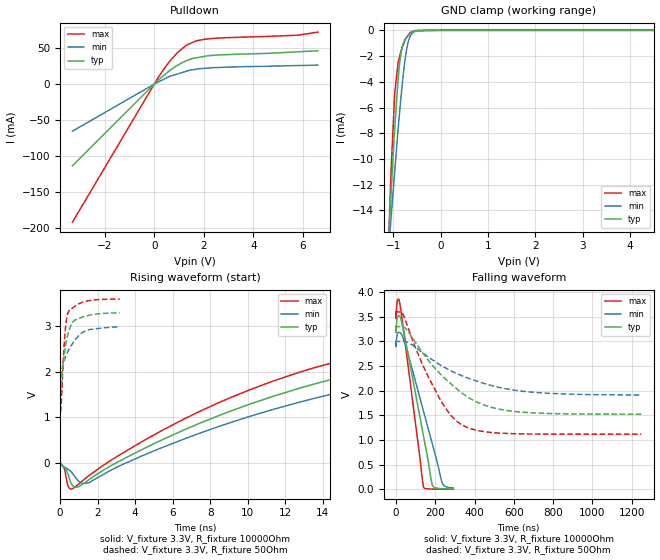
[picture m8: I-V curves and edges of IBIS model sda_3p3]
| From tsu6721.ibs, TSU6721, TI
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|   sda_3p3 Model
[Model]   sda_3p3
Model_type   I/O_open_drain
Polarity   Non-Inverting
Enable   Active-High
Vinl = 0.99
Vinh = 2.31
Vmeas = 1.65
Vref = 3.3
Cref = 35pF
Rref = 10000
|   typ   min   max
C_comp   1.333e-12   1.174e-12   1.472e-12
[Model spec]
Vinl   0.99   0.9   1.08
Vinh   2.31   2.1   2.52
[Voltage Range]   3.3   3   3.6
|Ambient Temperature   25   85   -40
|Junction Temperature
[Temperature Range]   27   125   -40
[Pullup Reference]   3.3   3   3.6
[Pulldown Reference]   0   0   0
[Power Clamp Reference]   3.3   3   3.6
[GND Clamp Reference]   0   0   0
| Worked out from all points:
|   slope of the pulldown table from 0 to 0.495 V, typ, clamps not added: 32.4 ohm
|   GND clamp passes 1 mA (typ) near -0.78 V on its own axis
|   falling waveform, V_fixture 3.3V, R_fixture 10000Ohm: 20-80 % time 93.2ns typ, 120ns min, 69.4ns max; typ from 3.3 V to 0.011 V
|   rising waveform, V_fixture 3.3V, R_fixture 10000Ohm: 20-80 % time 19.2ns typ, 21.2ns min, 17.1ns max; typ from 0.01 V to 3.3 V
|   falling waveform, V_fixture 3.3V, R_fixture 50Ohm: 20-80 % time 257ns typ, 332ns min, 180ns max; typ from 3.3 V to 1.53 V
|   rising waveform, V_fixture 3.3V, R_fixture 50Ohm: 20-80 % time 400ps typ, 813ps min, 226ps max; typ from 1.52 V to 3.3 V
[Pulldown]
|   Voltage   I(typ)   I(min)   I(max)
-3.3V     -113.6mA   -65.48mA   -192.1mA
205.2mV   6.801mA    3.646mA    11.59mA
633.6mV   19.16mA    10.93mA    32.29mA
946.8mV   26.41mA    14.25mA    44.23mA
1.246V    31.83mA    17.42mA    52.86mA
1.685V    36.59mA    20.75mA    60.14mA
2.149V    39.41mA    22.3mA     62.93mA
5.81V     45.04mA    25.89mA    68.18mA
6.6V      46.44mA    26.5mA     72.44mA
[GND Clamp]
|   Voltage   I(typ)   I(min)   I(max)
-3.3V     -194.3mA   -135.4mA   -293.9mA
-1.096V   -16.17mA   -17.09mA   -16.27mA
-1.044V   -12.67mA   -14.54mA   -10.88mA
-968.4mV  -7.687mA   -11.03mA   -4.931mA
-896.4mV  -3.773mA   -7.698mA   -2.481mA
-864.6mV  -2.548mA   -6.373mA   -2.035mA
-828.3mV  -1.609mA   -4.923mA   -1.535mA
-756mV    -742.2uA   -2.457mA   -821.6uA
-720mV    -555.8uA   -1.557mA   -551.1uA
-645mV    -280.8uA   -487.1uA   -190.1uA
-590.7mV  -81.64uA   -195.2uA   -95.61uA
6.6V      0A         0A         0A
[POWER Clamp]
|   Voltage   I(typ)   I(min)   I(max)
-3.3V     0A         0A         0A
-3.298V   0A         0A         0A
6.6V      0A         0A         0A
[Ramp]
R_load = 10000
|   typ   min   max
dV/dt_r   1.97429/1.9159e-08   1.79092/2.12873e-08   2.15634/1.70898e-08
dV/dt_f   1.97363/9.31778e-08   1.78798/1.20967e-07   2.1562/6.94673e-08
[Falling Waveform]
V_fixture = 3.3V
V_fixture_min = 3V
V_fixture_max = 3.6V
R_fixture = 10000Ohm
|   Time   V(typ)   V(min)   V(max)
0s        3.3V       3V         3.6V
175ps     3.182V     2.896V     3.465V
3.975ns   3.413V     3.09V      3.743V
9.05ns    3.507V     3.174V     3.849V
20.37ns   3.502V     3.178V     3.75V
46.82ns   3.053V     2.943V     2.969V
141.2ns   1.059V     1.571V     43.16mV
186.3ns   77.22mV    905.1mV    9.506mV
237.1ns   15.91mV    119mV      7.278mV
292.1ns   11.24mV    31.24mV    6.513mV
[Rising Waveform]
V_fixture = 3.3V
V_fixture_min = 3V
V_fixture_max = 3.6V
R_fixture = 10000Ohm
|   Time   V(typ)   V(min)   V(max)
0s        9.518mV    15.11mV    6.096mV
600ps     -466.6mV   -210.9mV   -585.2mV
1.075ns   -510.1mV   -439.7mV   -442.3mV
1.525ns   -380.6mV   -444.8mV   -292.7mV
6.625ns   721.7mV    521mV      962.6mV
11.28ns   1.447V     1.16V      1.781V
18.48ns   2.194V     1.849V     2.583V
26.4ns    2.686V     2.313V     3.082V
48.17ns   3.195V     2.85V      3.539V
84.75ns   3.296V     2.99V      3.599V
[Falling Waveform]
V_fixture = 3.3V
V_fixture_min = 3V
V_fixture_max = 3.6V
R_fixture = 50Ohm
|   Time   V(typ)   V(min)   V(max)
0s        3.3V       3V         3.6V
26.88ns   3.301V     3.001V     3.597V
36.9ns    3.296V     3V         3.54V
133.1ns   2.785V     2.779V     2.549V
234.1ns   2.308V     2.504V     1.763V
290.4ns   2.106V     2.385V     1.456V
348.5ns   1.918V     2.285V     1.283V
475.4ns   1.677V     2.119V     1.16V
611.1ns   1.578V     2.009V     1.13V
1.25us    1.526V     1.914V     1.12V
[Rising Waveform]
V_fixture = 3.3V
V_fixture_min = 3V
V_fixture_max = 3.6V
R_fixture = 50Ohm
|   Time   V(typ)   V(min)   V(max)
0s        1.525V     1.912V     1.12V
25ps      1.52V      1.899V     1.125V
50ps      1.623V     1.955V     1.246V
175ps     2.216V     2.191V     2.323V
275ps     2.533V     2.316V     2.919V
375ps     2.759V     2.415V     3.238V
475ps     2.913V     2.495V     3.345V
725ps     3.116V     2.659V     3.423V
1.325ns   3.22V      2.894V     3.545V
3.175ns   3.297V     2.99V      3.6V
